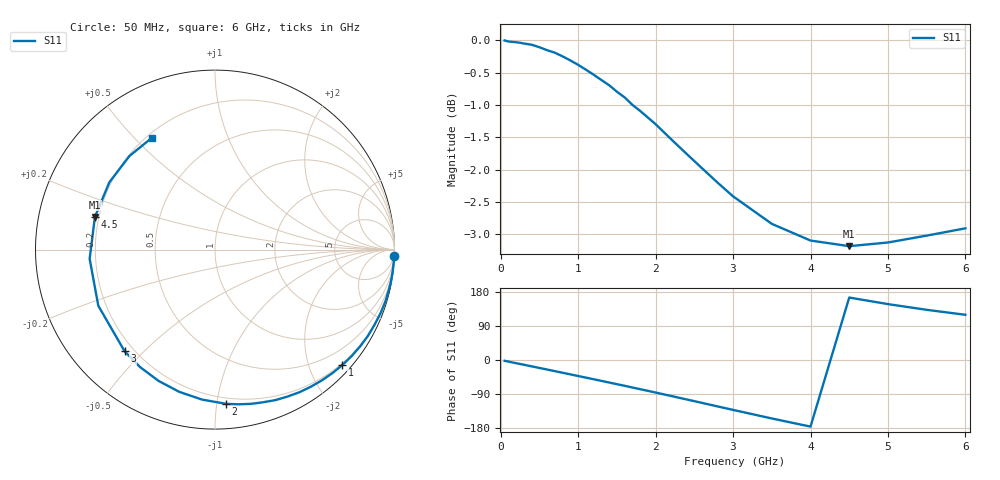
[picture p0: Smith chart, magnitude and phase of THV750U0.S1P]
! SIEMENS Discrete & RF Semiconductors
! BAS70
! Si Schottky Diode in SOT23
! VR = 0.75 V
! S-Parameters:  February  1997
# GHz  S  MA  R  50
!  f  S11
! GHz  MAG  ANG
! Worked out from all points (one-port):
!   34 points, 50 MHz to 6 GHz, reference 50 ohm
!   lowest |S11| = -3.2 dB at 4.5 GHz (marker M1), VSWR 5.52, Z = 9.21 + j6.45 ohm
!   |S11| at or under -10 dB: nowhere
!   S11 on the Smith chart (normalised r, x): 50 MHz: 0, -55; 1 GHz: 0.17, -2.58; 2 GHz: 0.16, -1.06; 3 GHz: 0.16, -0.44; 4.5 GHz: 0.18, +0.13; 6 GHz: 0.22, +0.56
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0.05  1 -2.1
0.25  0.9959 -10.5
0.4  0.9924 -16.8
0.5  0.988 -21.0
0.6  0.9827 -25.2
0.7  0.9784 -29.5
0.8  0.972 -33.7
0.9  0.965 -38.0
1  0.9575 -42.3
1.2  0.9408 -50.8
1.3  0.9319 -55.1
1.4  0.9234 -59.4
1.5  0.9128 -63.8
1.6  0.9036 -68.1
1.8  0.8821 -77.0
1.9  0.8718 -81.4
2  0.8615 -85.9
2.2  0.8388 -94.9
2.4  0.8172 -104.1
2.6  0.7964 -113.2
2.8  0.7764 -122.5
3  0.7577 -131.7
3.5  0.7215 -154.3
4  0.7003 -175.8
4.5  0.6933 164.8
5  0.6979 147.5
5.5  0.7065 132.4
6  0.7157 119.3
